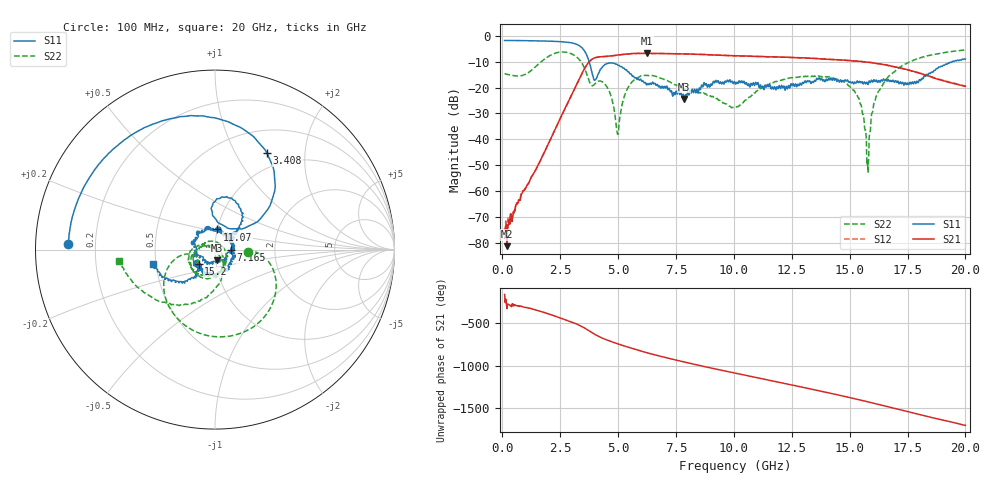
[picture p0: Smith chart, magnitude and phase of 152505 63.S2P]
!  2-Port S-parameters saved by WinCal
! VAR MeasName=S-Parameters (CALIBRATED_DATA) read from VNA (N5230C)
! VAR MeasDate=4/10/2015 9:35:13 AM
! VAR NAME=152505 63
! VAR FILENAME=152505 63.S2P
! VAR DATE=4/10/2015 9:35:13 AM
! VAR PHYS_PORTS=1,2
# Hz S DB R 50
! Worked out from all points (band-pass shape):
!   801 points, 100 MHz to 20 GHz, reference 50 ohm
!   highest |S21| = -6.70 dB at 6.244 GHz (marker M1); lowest = -81.4 dB at 199.5 MHz (marker M2)
!   |S21| within 3 dB of the highest: 3.783 GHz to 15.21 GHz (11.43 GHz wide, 120 % of centre); 15.24126 GHz to 15.26896 GHz (27.7 MHz wide, 0.182 % of centre)
!   lowest |S11| = -24.4 dB at 7.861 GHz (marker M3), VSWR 1.13, Z = 50.7 - j6.05 ohm
!   |S11| at or under -10 dB: 3.749 GHz to 19.44 GHz (15.69 GHz wide, 135 % of centre)
!   |S22| runs from -52.9 to -5.4 dB; largest |S21 - S12| = 0.0053
!   S11 on the Smith chart (normalised r, x): 100 MHz: 0.10, +0.02; 3.408 GHz: 0.79, +1.36; 7.165 GHz: 1.20, -0.01; 11.07 GHz: 1.00, +0.23; 15.2 GHz: 0.82, -0.14; 20 GHz: 0.48, -0.09
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1e8  -1.75 177.6  -78.29 -160.6  -74.55 -50.2  -14.59 -4.0
1.995e8  -1.76 175.2  -81.37 33.4  -72.59 74.4  -14.83 -5.7
2.09e9  -2.04 126.4  -39.90 -36.8  -39.83 -37.0  -7.43 -38.7
2.73675e9  -2.38 102.4  -27.55 -98.0  -27.59 -97.8  -6.30 -90.9
3.408375e9  -4.29 61.6  -15.08 -173.4  -15.09 -173.2  -10.14 -153.3
3.43325e9  -4.51 59.7  -14.64 -176.8  -14.64 -176.6  -10.48 -155.7
4.005375e9  -17.03 66.4  -8.45 89.2  -8.44 89.4  -18.53 -143.8
4.552625e9  -10.57 82.6  -7.86 21.0  -7.90 21.1  -20.26 177.7
4.9755e9  -11.16 61.7  -7.40 -19.7  -7.45 -19.9  -37.96 57.7
5.448125e9  -13.87 44.1  -6.97 -61.6  -6.95 -61.6  -19.70 -62.6
6.244125e9  -19.03 38.5  -6.70 -125.7  -6.76 -125.8  -15.35 -122.5
6.741625e9  -19.65 28.3  -6.78 -161.1  -6.80 -161.2  -16.01 -149.2
7.1645e9  -20.84 -2.4  -6.86 170.3  -6.85 170.5  -17.45 -165.1
7.861e9  -24.39 -80.1  -6.98 125.0  -6.94 125.3  -20.47 -178.9
1.005e10  -17.97 126.4  -7.66 -5.0  -7.69 -5.3  -27.48 47.2
1.106988e10  -18.93 83.0  -7.94 -63.0  -7.93 -63.1  -20.61 -47.6
1.338325e10  -17.64 -72.0  -8.69 163.9  -8.66 164.3  -15.54 -134.9
1.519912e10  -18.24 -138.3  -9.69 54.4  -9.62 54.3  -21.10 161.9
1.579612e10  -18.81 -138.8  -10.22 16.0  -10.14 16.2  -52.91 90.5
1.61195e10  -17.57 -138.2  -10.56 -5.5  -10.56 -5.7  -24.39 -56.9
1.669162e10  -17.13 -142.2  -11.46 -43.7  -11.48 -44.4  -15.59 -77.4
2e10  -8.95 -166.6  -19.51 98.4  -19.51 98.9  -5.37 -173.5
